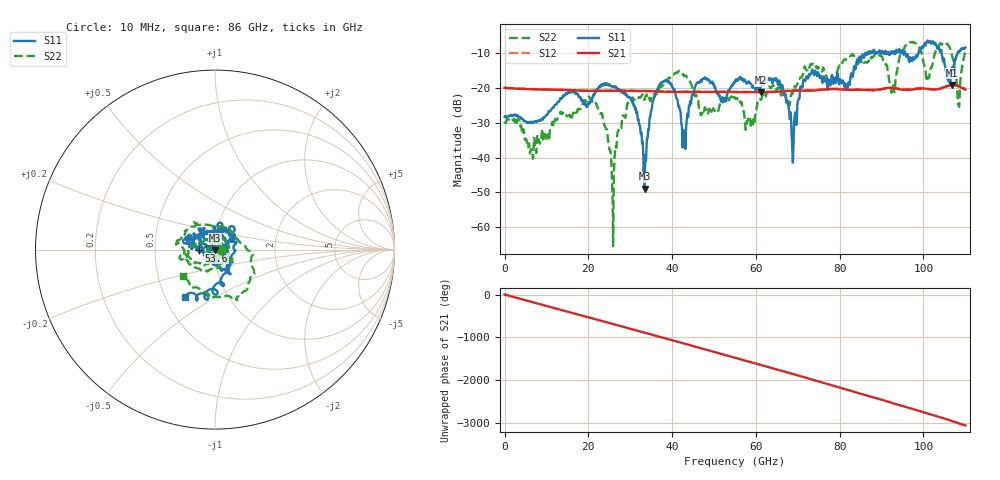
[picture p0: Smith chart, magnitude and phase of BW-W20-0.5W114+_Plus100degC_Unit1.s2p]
!Mini-Circuits Laboratory
!S-Parameters
!Model: BW-W20-0.5W114+
!Run / Lot / Date Code: QN2409253 /  / N/A
!Fixture:
!Network Analyzer: PNA-X N5242B - 423 4 ports (COM/DCOM);  Serial number: 74408
!Date: 3/8/2024 at 1:32:58 PM
!No.: Unit# 3 (U1  100C)
!Tested with:
# Hz  S  dB  R  50
!Frequency  S11 dB  S11 Deg  S21 dB  S21 Deg  S12 dB  S12 Deg  S22 dB  S22 Deg
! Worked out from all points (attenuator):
!   2208 points, 10 MHz to 110 GHz, reference 50 ohm
!   highest |S21| = -19.14 dB at 106.8 GHz (marker M1); lowest = -21.2 dB at 61.3 GHz (marker M2)
!   lowest |S11| = -49.0 dB at 33.45 GHz (marker M3), VSWR 1.01, Z = 49.9 - j0.348 ohm
!   |S11| at or under -10 dB: start of sweep to 86.04 GHz; 95.66 GHz to 98.78 GHz (3.117 GHz wide, 3.21 % of centre); 104.3 GHz to 108.1 GHz (3.791 GHz wide, 3.57 % of centre)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
!   |S22| runs from -65.5 to -6.8 dB; largest |S21 - S12| = 0.0042
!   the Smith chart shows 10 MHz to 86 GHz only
!   S11 on the Smith chart (normalised r, x): 10 MHz: 1.08, +0.00; 53.6 GHz: 0.84, -0.01; 86 GHz: 0.63, -0.37
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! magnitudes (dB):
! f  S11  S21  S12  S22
! 10 MHz  -28.3  -20.0  -19.9  -30.2
! 6.4 GHz  -29.7  -20.4  -20.3  -38.2
! 18.35 GHz  -23.7  -20.8  -20.7  -25.7
! 22.95 GHz  -19.3  -20.8  -20.8  -27.4
! 25.85 GHz  -19.5  -20.8  -20.8  -56.6
! 29.55 GHz  -22.6  -20.9  -20.8  -24.4
! 33.45 GHz  -49.0  -20.9  -20.9  -23.3
! 36.7 GHz  -19.7  -21.0  -20.9  -21.2
! 42.8 GHz  -33.4  -21.2  -21.1  -16.6
! 46.05 GHz  -18.4  -21.2  -21.1  -23.5
! 53.6 GHz  -21.1  -21.2  -21.1  -23.5
! 55.05 GHz  -18.3  -21.2  -21.1  -22.9
! 61.3 GHz  -18.9  -21.2  -21.2  -23.2
! 65.95 GHz  -20.3  -21.0  -20.9  -22.0
! 68.65 GHz  -36.4  -20.8  -20.7  -21.8
! 73.35 GHz  -14.9  -20.8  -20.7  -13.3
! 86 GHz  -10.2  -20.6  -20.6  -12.7
! 91.7 GHz  -10.1  -20.0  -20.0  -17.1
! 96.7 GHz  -11.9  -20.6  -20.3  -6.9
! 106.8 GHz  -14.2  -19.1  -19.1  -10.6
! 108.3 GHz  -9.7  -19.5  -19.3  -24.7
! 110 GHz  -8.4  -20.5  -20.2  -9.4
